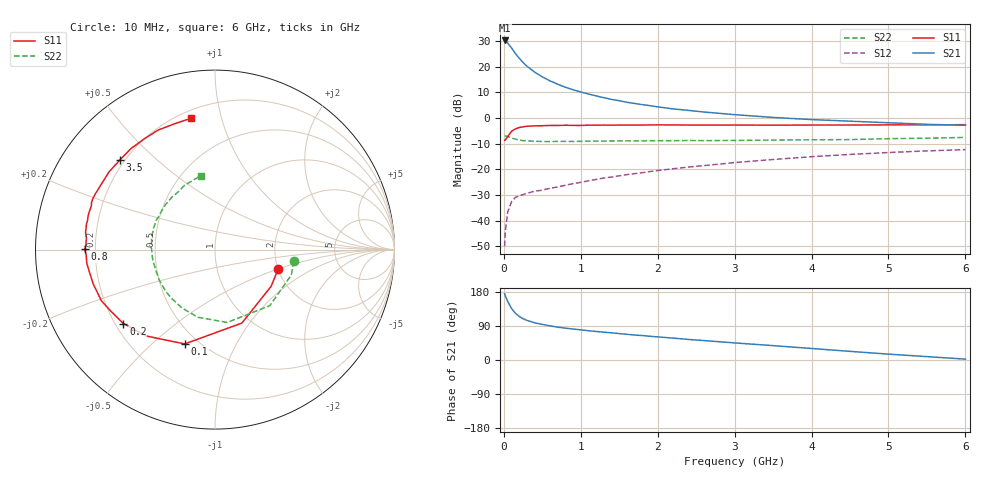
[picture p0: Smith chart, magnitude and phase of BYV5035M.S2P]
! SIEMENS Small Signal Semiconductors
! BFY420
! Si NPN RF SIEGET Grounded Emitter Transistor in MICRO-X
! VCE = 0.5 V  IC = 35 mA
! Common Emitter S-Parameters:  October  1996
# GHz  S  MA  R  50
!  f  S11  S21  S12  S22
! GHz  MAG  ANG  MAG  ANG  MAG  ANG  MAG  ANG
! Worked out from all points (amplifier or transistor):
!   36 points, 10 MHz to 6 GHz, reference 50 ohm
!   highest |S21| = 30.2 dB at 10 MHz (marker M1)
!   |S21| within 3 dB of that: start of sweep to 102 MHz
!   unconditionally stable (mu >= 1): start of sweep to 40.72 MHz; 467.7 MHz to end of sweep
!   at 250 MHz: K = 0.71, MSG = 25.7 dB, |S12| = -29.8 dB
!   at 1.4 GHz: K = 1.54, MAG = 10.8 dB, |S12| = -23.0 dB
!   at 6 GHz: K = 1.44, MAG = 0.8 dB, |S12| = -12.3 dB
!   S11 on the Smith chart (normalised r, x): 10 MHz: 2.00, -0.50; 100 MHz: 0.42, -0.64; 200 MHz: 0.23, -0.34; 800 MHz: 0.16, +0.00; 3.5 GHz: 0.18, +0.39; 6 GHz: 0.25, +0.81
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0.01  0.3683 -17.2  32.51 175.0  0.0032 96.0  0.4421 -8.4
0.02  0.3737 -33.2  32.13 168.6  0.0064 83.1  0.4484 -18.3
0.05  0.4359 -69.9  28.9 154.6  0.0148 68.2  0.437 -45.6
0.1  0.552 -107.8  23.25 135.9  0.0235 52.8  0.4115 -80.5
0.15  0.6151 -128.5  18.09 123.3  0.0285 45.1  0.3888 -104.2
0.2  0.6559 -141.1  14.68 115.0  0.0307 40.7  0.3739 -119.3
0.25  0.6748 -149.6  12.09 108.8  0.0324 38.7  0.364 -131.2
0.3  0.6938 -155.6  10.26 104.5  0.0343 38.4  0.3603 -139.2
0.4  0.7051 -164.2  7.867 98.4  0.0375 38.9  0.3537 -151.4
0.5  0.7099 -169.4  6.355 93.9  0.0396 39.7  0.35 -159.4
0.6  0.7183 -173.8  5.308 90.1  0.0429 41.4  0.3488 -164.8
0.7  0.7185 -177.6  4.57 86.6  0.0456 43.3  0.3515 -169.5
0.8  0.7256 179.7  3.99 84.1  0.0492 44.5  0.3513 -173.8
0.9  0.7199 177.7  3.559 81.7  0.0529 45.8  0.351 -177.2
1.1  0.7278 172.4  2.945 77.2  0.0601 47.6  0.3564 177.6
1.3  0.7305 168.9  2.496 73.4  0.0682 48.5  0.3558 172.4
1.6  0.7319 163.9  2.029 67.8  0.0793 48.5  0.3604 166.5
2.2  0.7353 154.9  1.51 57.8  0.1031 46.7  0.3633 156.8
3.5  0.7282 136.5  1.03 37.9  0.1561 37.1  0.3727 138.0
4.5  0.7324 122.4  0.87 22.8  0.196 26.2  0.3814 122.4
5.5  0.7367 107.1  0.756 8.9  0.2295 14.7  0.4056 107.3
6  0.7439 100.2  0.722 2.3  0.2431 9.1  0.42 100.8
